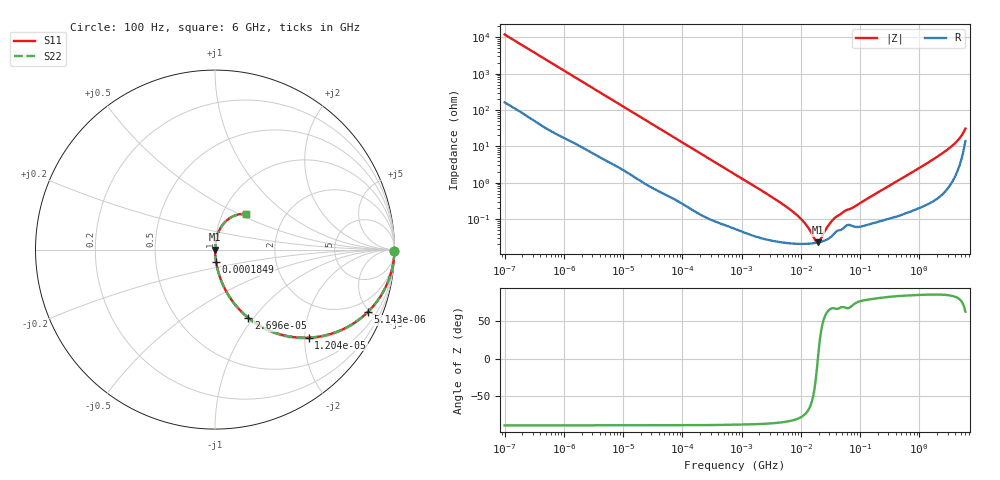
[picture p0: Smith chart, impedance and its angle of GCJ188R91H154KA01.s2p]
!Murata Part Number: GCJ188R91H154KA01
!These Parameters are Measured in Series Mode Connection
!Data Generated on Mar 13, 2026
!  o--ll--o
!Port1  Port2
!  o------o
!Operation Temp=25[degC], DC Bias Voltage=0[V]
!Freq. Start=100[Hz] Stop=6[GHz] 401[Steps]
# Hz S RI R 50
!Freq.(Hz) S11(Real) S11(Imag) S21(Real) S21(Imag) S12(Real) S12(Imag) S22(Real) S22(Imag)
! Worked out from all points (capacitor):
!   401 points, 100 Hz to 6 GHz, reference 50 ohm
!   read as one part in series: C = 132 nF near 109 Hz
!   lowest |Z| = 22.7 mohm at 19.46 MHz (marker M1)
!   series resonance near 19.39 MHz, so ESL is about 510 pH
!   S11 on the Smith chart (normalised r, x): 100 Hz: open; 5.143 kHz: 1.08, -4.84; 12.04 kHz: 1.04, -2.09; 26.96 kHz: 1.02, -0.94; 184.9 kHz: 1.00, -0.14; 6 GHz: 1.28, +0.55
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100  0.9998 -0.00831  0.000181 0.00831  0.000181 0.00831  0.9998 -0.00831
600  0.997 -0.0489  0.00304 0.0489  0.00304 0.0489  0.997 -0.0489
2008  0.9719 -0.1578  0.0281 0.1578  0.0281 0.1578  0.9719 -0.1578
5143  0.8501 -0.3486  0.1499 0.3486  0.1499 0.3486  0.8501 -0.3486
12041  0.5216 -0.4907  0.4784 0.4907  0.4784 0.4907  0.5216 -0.4907
26957  0.1856 -0.3801  0.8144 0.3801  0.8144 0.3801  0.1856 -0.3801
40335  0.0949 -0.2841  0.9051 0.2841  0.9051 0.2841  0.0949 -0.2841
82567  0.0266 -0.1511  0.9734 0.1511  0.9734 0.1511  0.0266 -0.1511
184852  0.00632 -0.0697  0.9937 0.0697  0.9937 0.0697  0.00632 -0.0697
774597  0.000823 -0.017  0.9992 0.017  0.9992 0.017  0.000823 -0.017
6948629  0.000216 -0.0017  0.9998 0.0017  0.9998 0.0017  0.000216 -0.0017
1.137099e7  0.000208 -0.000786  0.9998 0.000786  0.9998 0.000786  0.000208 -0.000786
1.555665e7  0.000214 -0.000313  0.9998 0.000313  0.9998 0.000313  0.000214 -0.000313
1.779312e7  0.00022 -0.000122  0.9998 0.000122  0.9998 0.000122  0.00022 -0.000122
1.946e7  0.000227 4.9e-06  0.9998 -4.9e-06  0.9998 -4.9e-06  0.000227 4.9e-06
2.128304e7  0.000234 0.000132  0.9998 -0.000132  0.9998 -0.000132  0.000234 0.000132
3.045065e7  0.0003 0.000667  0.9997 -0.000667  0.9997 -0.000667  0.0003 0.000667
3.80911e7  0.000427 0.00101  0.9996 -0.00101  0.9996 -0.00101  0.000427 0.00101
3.124326e8  0.00108 0.00818  0.9989 -0.00818  0.9989 -0.00818  0.00108 0.00818
2.562649e9  0.0096 0.0669  0.9904 -0.0669  0.9904 -0.0669  0.0096 0.0669
4.385646e9  0.0381 0.1322  0.9619 -0.1322  0.9619 -0.1322  0.0381 0.1322
6e9  0.1715 0.2001  0.8285 -0.2001  0.8285 -0.2001  0.1715 0.2001
